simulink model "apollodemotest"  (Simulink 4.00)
settings: Solver=ode45  SolverMode=SingleTasking  StartTime=0  StopTime=100  MaxStep=0.01  RelTol=1e-6  AbsTol=1e-6
undefined symbols (not defined in the file or in its folder): Reference

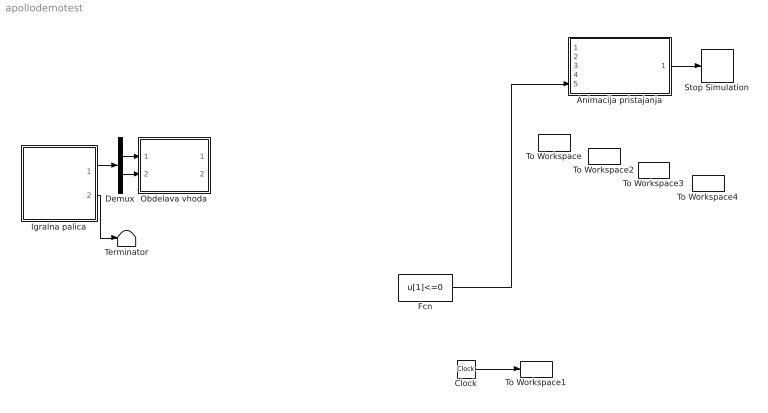
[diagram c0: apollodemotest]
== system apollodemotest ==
  Animacija pristajanja : Subsystem
  Clock : Clock
  Demux : Demux  Outputs=2  BusSelectionMode=off
  Fcn : Fcn  Expr=u[1]<=0
  Igralna palica : Subsystem  mask(Palica){dT__S_fun=0.1}
      mask prompts: dT__S_fun "Cas vzorcenja"
      mask help: Na prvem vhodu dobimo x in y koordinato palice (v dvodimenzionalnem vektorju), na drugem pa stanje gumbov (v stiridimenzionalnem vektorju). Ce je gumb pritisnjen, se na pripadajocem izhodu pojavi 0, sicer pa 1.
  Obdelava vhoda : Subsystem
  Stop Simulation : Stop
  Terminator : Terminator
  To Workspace : ToWorkspace  VariableName=x  SampleTime=0.1  SaveFormat=Array
  To Workspace1 : ToWorkspace  VariableName=t  SampleTime=0.1  SaveFormat=Array
  To Workspace2 : ToWorkspace  VariableName=y  SampleTime=0.1  SaveFormat=Array
  To Workspace3 : ToWorkspace  VariableName=v_y  SampleTime=0.1  SaveFormat=Array
  To Workspace4 : ToWorkspace  VariableName=m  SampleTime=0.1  SaveFormat=Array
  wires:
  Clock/1 -> To Workspace1/1
  ? -> To Workspace/1, Animacija pristajanja/1(x)
  ? -> To Workspace4/1, Animacija pristajanja/3(m)
  ? -> To Workspace3/1, Animacija pristajanja/4(v_y)
  Igralna palica/1(Out1) -> Demux/1
  Demux/1 -> Obdelava vhoda/1(In1)
  Demux/2 -> Obdelava vhoda/2(In2)
  Obdelava vhoda/1(Out1) -> ?
  Obdelava vhoda/2(Out2) -> ?
  ? -> To Workspace2/1, Animacija pristajanja/2(y), Fcn/1
  Animacija pristajanja/1(konec) -> Stop Simulation/1
  Igralna palica/2(Out2) -> Terminator/1
  Fcn/1 -> Animacija pristajanja/5(hit)

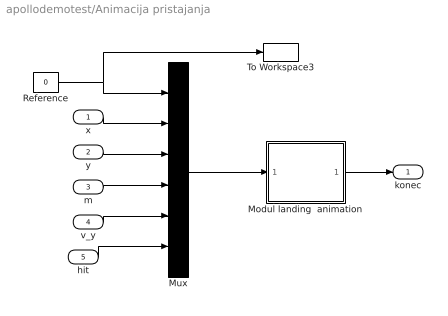
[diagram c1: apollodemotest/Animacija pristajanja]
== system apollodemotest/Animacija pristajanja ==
  x : Inport  Port=1  LatchInput=off
  y : Inport  Port=2  LatchInput=off
  m : Inport  Port=3  LatchInput=off
  v_y : Inport  Port=4  LatchInput=off
  hit : Inport  Port=5  LatchInput=off
  Modul landing  animation : Subsystem  mask(Modul landing plot){RefBlock=Reference}
      mask prompts: RefBlock "DC reference signal block name:"
      mask help: Modul landing plot
  Mux : Mux  Inputs=6
  Reference : Constant  Value=0
  To Workspace3 : ToWorkspace  VariableName=ref  SampleTime=0.1  SaveFormat=Array
  konec : Outport  Port=1
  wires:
  Mux/1 -> Modul landing  animation/1(in_1)
  x/1 -> Mux/2
  y/1 -> Mux/3
  m/1 -> Mux/4
  v_y/1 -> Mux/5
  Reference/1 -> Mux/1, To Workspace3/1
  hit/1 -> Mux/6
  Modul landing  animation/1(Out_1) -> konec/1

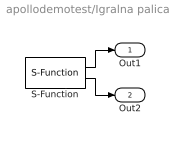
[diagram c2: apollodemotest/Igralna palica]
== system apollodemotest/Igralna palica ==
  S-Function : S-Function  FunctionName=palica  Parameters=dT__S_fun  PortCounts=[]  SFunctionModules=''
  Out1 : Outport  Port=1  InitialOutput=0
  Out2 : Outport  Port=2  InitialOutput=0
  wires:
  S-Function/2 -> Out2/1
  S-Function/1 -> Out1/1

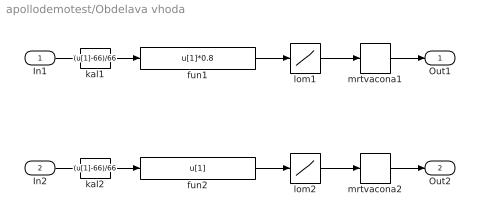
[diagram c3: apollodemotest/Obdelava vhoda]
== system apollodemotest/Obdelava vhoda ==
  In1 : Inport  Port=1  LatchInput=off
  In2 : Inport  Port=2  LatchInput=off
  fun1 : Fcn  Expr=u[1]*0.8
  fun2 : Fcn  Expr=u[1]
  kal1 : Fcn  Expr=(u[1]-66)/66
  kal2 : Fcn  Expr=(u[1]-66)/66
  lom1 : Lookup  InputValues=[-1 -0.5 0.5 1]  OutputValues=[-2.8 -0.4 0.4 2.8]
  lom2 : Lookup  InputValues=[-1 -0.5 0.5 1]  OutputValues=[-2.8 -0.4 0.4 2.8]
  mrtvacona1 : DeadZone  LowerValue=-0.05  UpperValue=0.05  SaturateOnIntegerOverflow=on  LinearizeAsGain=on
  mrtvacona2 : DeadZone  LowerValue=0  UpperValue=0  SaturateOnIntegerOverflow=on  LinearizeAsGain=on
  Out1 : Outport  Port=1
  Out2 : Outport  Port=2
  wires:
  In1/1 -> kal1/1
  In2/1 -> kal2/1
  kal1/1 -> fun1/1
  kal2/1 -> fun2/1
  mrtvacona1/1 -> Out1/1
  mrtvacona2/1 -> Out2/1
  lom1/1 -> mrtvacona1/1
  lom2/1 -> mrtvacona2/1
  fun1/1 -> lom1/1
  fun2/1 -> lom2/1

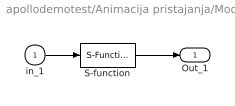
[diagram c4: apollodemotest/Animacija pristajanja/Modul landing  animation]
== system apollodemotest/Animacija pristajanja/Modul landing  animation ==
  in_1 : Inport  Port=1  LatchInput=off
  S-function : S-Function  FunctionName=modulan  Parameters=RefBlock  PortCounts=[]  SFunctionModules=''
  Out_1 : Outport  Port=1
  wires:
  in_1/1 -> S-function/1
  S-function/1 -> Out_1/1
